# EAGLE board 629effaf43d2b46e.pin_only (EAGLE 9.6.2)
REV: B

Size 17.78 x 20.7 mm. Coordinates in mm from the lower left corner, seen from the top.
Outline: 17.78,18.16 17.78,2.54 arc-90 15.24,0 2.54,0 arc-90 0,2.54 0,18.16 arc-90 2.54,20.7 15.24,20.7 arc-90 17.78,18.16
Copper layers (1*16): Top 0.035mm / dielectric 1.5mm / Bottom 0.035mm
Design rules "adafruit 6-6 *": minimum track width 6mil, minimum drill 15.5mil, track to track 6mil, track to pad 6mil, pad to pad 6mil, via to via 6mil, smd to smd 6mil, copper to edge 10mil, drill to drill 8mil, minimum pad ring 10mil, minimum via ring 8mil, stop-mask expansion 2mil, vias tented up to drill 20mil, thermal gap 10mil
Net classes: 1 power: width 0.254 mm; 2 gnd: width 0.254 mm

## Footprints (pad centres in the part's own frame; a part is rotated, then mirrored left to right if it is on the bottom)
0805-NO = smd 1.24 x 1.5: 1 -0.95,0; 2 0.95,0
_0402NO = smd 0.6 x 0.6: 1 -0.508,0; 2 0.508,0
JST_SH4_SKINNY = smd 0.5 x 1.55: 1 -1.5,2.514; 2 -0.5,2.514; 3 0.5,2.514; 4 1.5,2.514 | smd 1.2 x 1.8: MT1 -2.8,-1.386; MT2 2.8,-1.386
SOD-323_MINI = smd 0.9 x 0.8: A 1.07,0; C -1.07,0
TESTPOINT_MINUS_1X3MM = smd 0.5 x 0.5: P$1 0.8,-0.05
1X07_CASTEL = drill 1 pad 1.778: 1 -7.62,0; 2 -5.08,0; 3 -2.54,0; 4 0,0; 5 2.54,0; 6 5.08,0; 7 7.62,0 | drill 1 pad 1.778 long: 1C -7.62,-1.27; 2C -5.08,-1.27; 3C -2.54,-1.27; 4C 0,-1.27; 5C 2.54,-1.27; 6C 5.08,-1.27; 7C 7.62,-1.27
_0402 = smd 0.6 x 0.6: 1 -0.508,0; 2 0.508,0
SK6805_1515 = smd 0.5 x 0.5: 1 -0.5,-0.45; 2 0.5,-0.45; 3 0.5,0.45; 4 -0.5,0.45
BTN_KMR2_4.6X2.8 = smd 0.9 x 0.9: A 2.05,0.8; A' -2.05,0.8; B 2.05,-0.8; B' -2.05,-0.8
BTN_KMR2_SLIM = smd 0.9 x 0.85: A 2.05,0.825; A' -2.05,0.825; B 2.05,-0.825; B' -2.05,-0.825
_0603MP_TWO6MIL = smd 0.8 x 0.8: 1 -0.787,0; 2 0.787,0
B1,27 = smd 1.27 x 1.27: TP 0,0
SOT23-5 = smd 0.55 x 1.2: 1 -0.95,-1.3; 2 0,-1.3; 3 0.95,-1.3; 4 0.95,1.3; 5 -0.95,1.3
QFN32_5MM = smd 0.81 x 0.27: 1 -2.45,1.75; 2 -2.45,1.25; 3 -2.45,0.75; 4 -2.45,0.25; 5 -2.45,-0.25; 6 -2.45,-0.75; 7 -2.45,-1.25; 8 -2.45,-1.75; 17 2.45,-1.75; 18 2.45,-1.25; 19 2.45,-0.75; 20 2.45,-0.25; 21 2.45,0.25; 22 2.45,0.75; 23 2.45,1.25; 24 2.45,1.75 | smd 0.27 x 0.81: 9 -1.75,-2.45; 10 -1.25,-2.45; 11 -0.75,-2.45; 12 -0.25,-2.45; 13 0.25,-2.45; 14 0.75,-2.45; 15 1.25,-2.45; 16 1.75,-2.45; 25 1.75,2.45; 26 1.25,2.45; 27 0.75,2.45; 28 0.25,2.45; 29 -0.25,2.45; 30 -0.75,2.45; 31 -1.25,2.45; 32 -1.75,2.45 | smd 3 x 3: 33 0,0
FIDUCIAL_1MM = smd 1 x 1: 1 0,0
TESTPOINT_PLUS_1X3MM = smd 0.5 x 0.5: P$1 0.8,-0.05
ANT_2450AT18B100 = smd 1.6 x 1.8: FP -1.4,0; NC 1.4,0
USB_C_CUSB31-CFM2AX-01-X = smd 0.575 x 1.15: A1B12 -3.2,3.545; A4B9 -2.4,3.545; B1A12 3.2,3.545; B4A9 2.4,3.545 | smd 0.275 x 1.15: A5 -1.25,3.545; A6 -0.25,3.545; A7 0.25,3.545; A8 1.25,3.545; B5 1.75,3.545; B6 0.75,3.545; B7 -0.75,3.545; B8 -1.75,3.545 | drill 0.6 pad 1 long: M1 -4.32,2.97; M2 4.32,2.97; M3 -4.32,-1.21; M4 4.32,-1.21 | hole 0.65: 2.89,2.47; -2.89,2.47
CRYSTAL_2X1.6 = smd 0.75 x 0.7: 1 -0.675,-0.5; 2 0.675,-0.5; 3 0.675,0.5; 4 -0.675,0.5

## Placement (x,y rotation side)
C1  22uF  [0805-NO]  11.94,12.74 180 top
C2  1uF  [_0402NO]  6.86,13.7 0 bottom
C3  1uF  [_0402NO]  3.3,15.94 270 bottom
C4  0.1uF  [_0402NO]  6.86,12.62 0 bottom
C6  22uF  [0805-NO]  13.42,9.8 90 top
C7  TBD  [_0402NO]  5.05,6.49 0 bottom
C8  22uF  [0805-NO]  10.45,6.93 180 top
C9  TBD  [_0402NO]  5.07,5.3 0 bottom
C10  0.1uF  [_0402NO]  3.94,7.92 0 bottom
C11  1uF  [_0402NO]  14.05,7.94 270 bottom
C14  0.1uF  [_0402NO]  14.24,9.84 270 bottom
C15  1uF  [_0402NO]  9.35,4.38 270 bottom
C16  0.01uF  [_0402NO]  8.27,4.38 270 bottom
C17  16pF  [_0402NO]  10.29,1.98 270 bottom
C18  16pF  [_0402NO]  14.01,1.22 180 bottom
CONN1  STEMMA_I2C_QTSKINNY  [JST_SH4_SKINNY]  11.07,2.58 0 top
D1  NSR0320  [SOD-323_MINI]  10.82,16.43 0 bottom
D2  NSR0320  [SOD-323_MINI]  14.33,17.21 90 bottom
GND  [TESTPOINT_MINUS_1X3MM]  6.99,18.92 270 bottom
JP1  [1X07_CASTEL]  1.27,10.35 270 top
JP3  [1X07_CASTEL]  16.51,10.35 90 top
L1  2nH  [_0402]  6.02,7.92 180 bottom
L2  0 ohm  [_0402]  6.77,5.94 90 bottom
LED1  WS2812B_SK6805_1515  [SK6805_1515]  13.07,6.97 180 top
Q1  BOOT0  [BTN_KMR2_4.6X2.8]  6.1,11.05 180 top
Q2  reset  [BTN_KMR2_SLIM]  6.1,7.11 0 top
R1  10K  [_0402NO]  3.75,17.46 0 bottom
R2  10K  [_0402NO]  9.22,2.45 270 bottom
R3  0  [_0402NO]  11.96,3.89 0 bottom
R4  1k  [_0402NO]  14.22,2.54 270 bottom
R5  5.1K  [_0402NO]  7.3,13.11 0 top
R6  5.1K  [_0402NO]  9.27,12.93 0 top
R7  10K  [_0603MP_TWO6MIL]  9.12,13.65 180 bottom
SWC1  TPB1,27  [B1,27]  2.54,19.56 0 bottom
SWC2  TPB1,27  [B1,27]  14.5,13.91 0 bottom
U1  AP2112K-3.3  [SOT23-5]  10.86,9.87 180 top
U2  ESP32-C3FH4  [QFN32_5MM]  10.54,8.32 180 bottom
U$3  [QTPYC3_TOP]  0,0 0 top
U$6  FIDUCIAL_1MM  [FIDUCIAL_1MM]  6.2,19.49 0 top
U$8  FIDUCIAL_1MM  [FIDUCIAL_1MM]  10.86,0.76 0 top
U$12  [PCBFEAT-REV-040]  13.91,4.99 0 bottom
U$18  [QTPYC3_BOT]  17.78,0 0 bottom
VBAT  [TESTPOINT_PLUS_1X3MM]  10.79,18.92 270 bottom
X1  2.4GHz  [ANT_2450AT18B100]  4.83,1.33 180 top
X6  USB TYPE C  [USB_C_CUSB31-CFM2AX-01-X]  8.89,17.91 180 top
Y1  40MHz  [CRYSTAL_2X1.6]  11.87,2.2 270 bottom

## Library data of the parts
C1-C4 C6-C11 C14-C18 CONN1 D1 D2 GND JP1 JP3 L1 L2 LED1 R1-R7 U$12 VBAT Y1 = microbuilder
Q1 Q2 X6 = adafruit_electromech
SWC1 SWC2 = testpad
U1 = adafruit_power
U2 = adafruit_wireless; DESCRIPTION: Bluetooth, WiFi 802.11b/g/n, Bluetooth v5.0 Transceiver Module 2.402GHz ~ 2.48GHz Antenna Not Included Surface Mount; DIGI-KEY_PART_NUMBER: 1904-ESP32-C3FH4CT-ND; MF: Espressif Systems; MP: ESP32-C3FH4; PACKAGE: VFQFN-32 Espressif Systems; PURCHASE-URL: https://pricing.snapeda.com/search/part/ESP32-C3FH4/?ref=eda
U$3 U$18 = itsy_silks
U$6 U$8 = microbuilder; BOM: EXCLUDE
X1 = adafruit_wireless

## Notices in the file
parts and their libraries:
microbuilder: This work is placed in the public domain, and may be freely used for commercial and non-commercial work with the following conditions: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
